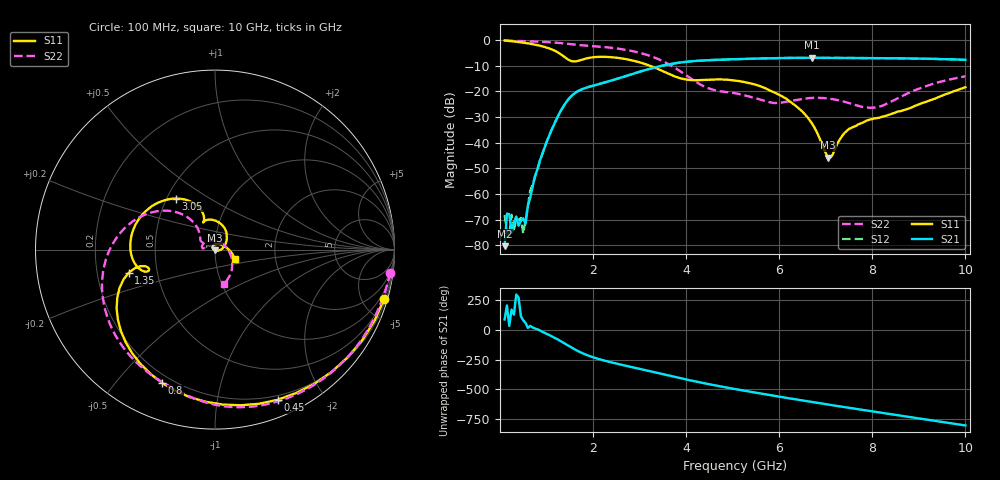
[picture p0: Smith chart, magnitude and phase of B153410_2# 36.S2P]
!  2-Port S-parameters saved by WinCal
! VAR MeasName=S-Parameters (CALIBRATED_DATA) read from VNA (N5245A)
! VAR MeasDate=2016-12-23 10:01:12
! VAR NAME=B153410_2# 36
! VAR FILENAME=B153410_2# 36.S2P
! VAR DATE=2016-12-23 10:01:12
! VAR PHYS_PORTS=1,2
# Hz S DB R 50
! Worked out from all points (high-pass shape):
!   199 points, 100 MHz to 10 GHz, reference 50 ohm
!   highest |S21| = -6.89 dB at 6.7 GHz (marker M1); lowest = -80.3 dB at 100 MHz (marker M2)
!   |S21| within 3 dB of the highest: 3.507 GHz to end of sweep
!   lowest |S11| = -45.8 dB at 7.05 GHz (marker M3), VSWR 1.01, Z = 49.9 - j0.495 ohm
!   |S11| at or under -10 dB: 3.223 GHz to end of sweep
!   |S22| runs from -26.4 to -0.1 dB; largest |S21 - S12| = 0.0033
!   S11 on the Smith chart (normalised r, x): 100 MHz: 0.45, -7.01; 450 MHz: 0.16, -1.49; 800 MHz: 0.16, -0.67; 1.35 GHz: 0.34, -0.12; 3.05 GHz: 0.56, +0.36; 10 GHz: 1.24, -0.13
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1e8  -0.15 -16.2  -80.35 89.4  -68.21 126.1  -0.13 -7.5
1.5e8  -0.24 -24.0  -67.67 -152.6  -74.71 -17.7  -0.18 -10.9
2e8  -0.33 -31.5  -67.88 34.6  -76.40 75.9  -0.22 -14.3
2.5e8  -0.42 -39.0  -75.00 171.8  -68.10 6.4  -0.25 -17.7
3e8  -0.52 -46.3  -71.15 130.3  -74.56 146.5  -0.28 -21.0
4.5e8  -0.85 -67.4  -70.52 116.3  -69.33 51.6  -0.37 -31.0
5e8  -0.98 -74.1  -69.49 82.2  -75.50 40.1  -0.39 -34.2
5.5e8  -1.12 -80.7  -71.62 59.9  -70.20 3.5  -0.42 -37.5
6.5e8  -1.42 -93.5  -61.46 35.4  -58.74 37.5  -0.48 -44.1
8e8  -1.94 -111.6  -50.62 6.7  -50.86 9.6  -0.59 -53.9
1.35e9  -6.08 -165.0  -26.25 -104.1  -26.23 -104.0  -1.24 -89.3
1.75e9  -7.71 -162.7  -19.25 167.8  -19.22 168.1  -2.00 -111.7
3.05e9  -8.93 127.3  -12.09 27.2  -12.07 27.1  -5.17 172.9
3.4e9  -11.30 113.1  -10.35 -4.3  -10.34 -4.4  -7.39 152.1
4.25e9  -15.62 113.7  -8.06 -78.9  -8.07 -79.0  -16.68 130.0
5.05e9  -15.75 91.1  -7.43 -139.4  -7.45 -139.3  -20.72 148.9
6.1e9  -22.30 35.0  -6.97 150.0  -6.98 150.1  -24.19 171.3
6.7e9  -32.40 -8.9  -6.89 111.5  -6.90 111.5  -22.56 167.7
7.05e9  -45.84 -103.3  -6.93 89.5  -6.93 89.7  -22.78 152.7
7.5e9  -34.60 141.0  -6.94 62.3  -6.96 62.2  -24.53 122.9
8.35e9  -29.10 64.9  -7.08 11.3  -7.07 11.3  -24.44 17.4
1e10  -18.35 -24.5  -7.69 -87.0  -7.71 -86.7  -14.10 -74.9
